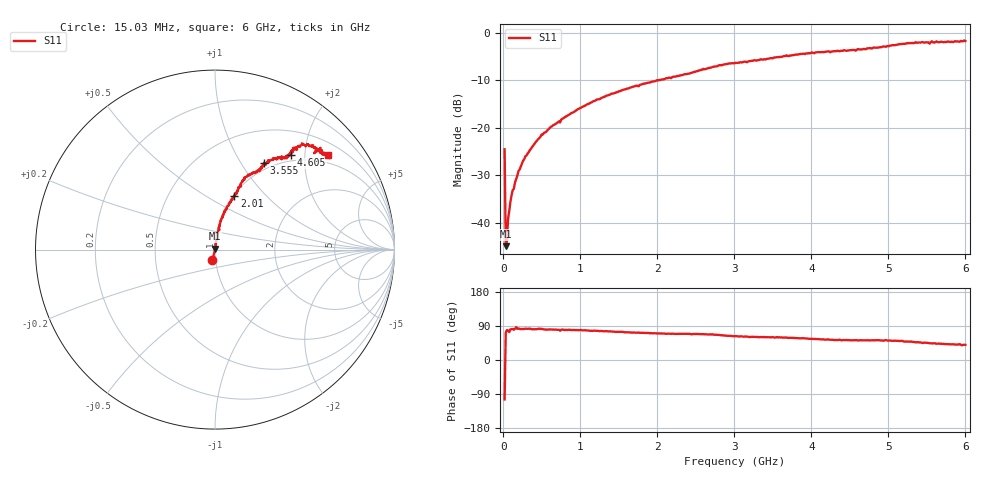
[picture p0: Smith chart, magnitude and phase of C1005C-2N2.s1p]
!	Network	Analyzer	HP8753E.07.74:	Oct	30	2002	Serial	No.	JP38451487
!	Hewlett-Packard
!	7	Sep	2009	8:17:41
!	Frequency	S11
#	HZ	S	RI	R	50
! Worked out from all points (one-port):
!   400 points, 15.03 MHz to 6 GHz, reference 50 ohm
!   lowest |S11| = -44.9 dB at 30.03 MHz (marker M1), VSWR 1.01, Z = 50.2 + j0.542 ohm
!   |S11| at or under -10 dB: start of sweep to 1.991 GHz; 2.008062 GHz to 2.010978 GHz (2.916 MHz wide, 0.145 % of centre)
!   S11 on the Smith chart (normalised r, x): 15.03 MHz: 0.97, -0.11; 2.01 GHz: 1.02, +0.67; 3.555 GHz: 0.91, +1.27; 4.605 GHz: 0.89, +1.73; 6 GHz: 0.79, +2.54
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1.502992e7  -0.0143 -0.0576
3.002985e7  0.0017 0.0054
4.502978e7  0.00124 0.00634
6.00297e7  0.00228 0.0108
9.002955e7  0.00265 0.0163
1.200294e8  0.00317 0.0218
1.350293e8  0.00401 0.0224
1.95029e8  0.00421 0.0347
2.850286e8  0.00639 0.0498
4.950275e8  0.011 0.0842
7.650262e8  0.0203 0.123
1.215024e9  0.0443 0.194
1.515022e9  0.0659 0.234
2.01002e9  0.108 0.297
2.265019e9  0.125 0.329
3.015015e9  0.219 0.431
3.555012e9  0.274 0.484
3.765011e9  0.305 0.496
4.515007e9  0.407 0.517
4.605007e9  0.424 0.526
4.965005e9  0.434 0.566
5.265004e9  0.52 0.585
5.445003e9  0.567 0.564
5.535002e9  0.552 0.537
5.565002e9  0.588 0.567
5.595002e9  0.564 0.551
5.625002e9  0.596 0.554
6e9  0.63 0.526
